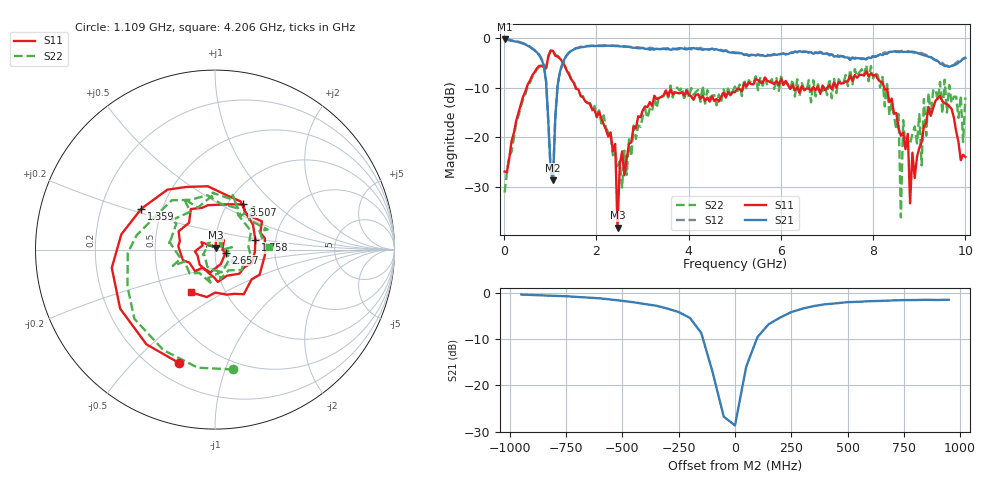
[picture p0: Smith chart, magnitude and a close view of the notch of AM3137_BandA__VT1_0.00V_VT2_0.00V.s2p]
! Date/Time: Tue, Nov 13, 2018 4:47 PM
! Network Analyzer: Agilent Technologies E8364B Rev: A.07.50.67
! Sweep from 0.010 to 10.000 GHz, 201 Points, Sweep Type: LIN
! Power Supply: -0.000 V, 0.000 A
# Hz S DB R 50
!freq MagS11 AngS11 MagS21 AngS21 MagS12 AngS12 MagS22 AngS22
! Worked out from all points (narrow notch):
!   201 points, 10 MHz to 10 GHz, reference 50 ohm
!   highest |S21| = -0.24 dB at 10 MHz (marker M1); lowest = -28.6 dB at 1.059 GHz (marker M2)
!   notch at M2: 25.8 dB deep, 160 MHz wide at half that depth
!   lowest |S11| = -38.1 dB at 2.458 GHz (marker M3), VSWR 1.03, Z = 50.4 + j1.16 ohm
!   |S11| at or under -10 dB: start of sweep to 486.9 MHz; 1.552 GHz to 5.177 GHz (3.625 GHz wide, 108 % of centre); 8.239 GHz to end of sweep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
!   |S22| runs from -36.1 to -2.5 dB; largest |S21 - S12| = 0.034
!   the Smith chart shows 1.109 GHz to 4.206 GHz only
!   S11 on the Smith chart (normalised r, x): 1.109 GHz: 0.30, -0.69; 1.359 GHz: 0.38, +0.22; 1.758 GHz: 1.57, +0.18; 2.657 GHz: 1.12, -0.04; 3.507 GHz: 1.18, +0.65; 4.206 GHz: 0.69, -0.36
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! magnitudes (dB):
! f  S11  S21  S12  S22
! 10 MHz  -26.9  -0.2  -0.2  -31.1
! 859.2 MHz  -5.9  -5.5  -5.4  -5.9
! 1.059 GHz  -2.6  -28.6  -28.4  -2.5
! 1.109 GHz  -3.6  -16.0  -15.9  -3.4
! 1.359 GHz  -6.6  -3.5  -3.4  -6.3
! 1.708 GHz  -11.9  -1.8  -1.7  -11.7
! 1.758 GHz  -12.7  -1.7  -1.6  -12.7
! 2.408 GHz  -21.3  -1.6  -1.5  -22.7
! 2.458 GHz  -38.1  -1.6  -1.5  -25.7
! 2.657 GHz  -24.2  -1.7  -1.7  -27.5
! 3.357 GHz  -12.0  -2.2  -2.3  -11.8
! 3.507 GHz  -10.5  -2.3  -2.1  -10.6
! 4.206 GHz  -11.3  -2.2  -2.1  -10.4
! 5.005 GHz  -10.9  -3.0  -2.9  -9.8
! 6.703 GHz  -9.9  -3.2  -2.9  -8.5
! 8.352 GHz  -12.9  -2.8  -2.8  -15.5
! 8.551 GHz  -18.1  -2.8  -2.7  -15.3
! 8.601 GHz  -19.7  -2.7  -2.6  -36.1
! 8.651 GHz  -19.1  -2.8  -2.6  -16.5
! 8.801 GHz  -33.3  -2.8  -2.7  -21.3
! 9.451 GHz  -11.7  -5.1  -4.9  -8.8
! 10 GHz  -23.9  -4.0  -3.9  -11.9
